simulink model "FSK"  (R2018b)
settings: Solver=VariableStepAuto  StartTime=0.0  StopTime=20  FixedStep=1e-5  RelTol=1e-3
libraries: commdigbbndfm2 x2, commchan3 x1, commrandsrc3 x1, dspsrcs4 x1

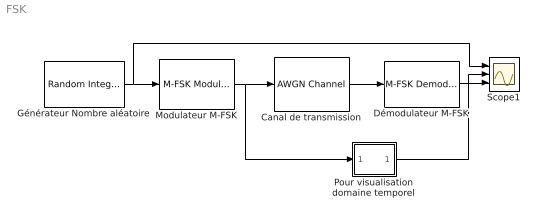
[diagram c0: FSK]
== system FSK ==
  Canal de transmission : commchan3/AWGN Channel  InputProcessing=Columns as channels (frame based)  seed=67  noiseMode="Signal to noise ratio  (Eb/No)"  EbNodB=10  EsNodB=10  SNRdB=10  bitsPerSym=1  Ps=1  Tsym=1  variance=1
  Démodulateur M-FSK : commdigbbndfm2/M-FSK Demodulator Baseband  M=4  OutType=Integer  Dec=Binary  freqSep=10  numSamp=100000  RateOptions=Enforce single-rate processing  outDataType=double
  Générateur Nombre aléatoire : commrandsrc3/Random Integer Generator  SetSize=4  SeedSource=Auto  Seed=0  SampleTime=1  SamplesPerFrame=1  OutputDataType=double  SimulateUsing=Interpreted execution
  Modulateur M-FSK : commdigbbndfm2/M-FSK Modulator Baseband  M=4  InType=Integer  Enc=Binary  freqSep=10  phaseType=Continuous  numSamp=100000  RateOptions=Enforce single-rate processing  outDataType=double
  Pour visualisation domaine temporel : Subsystem
  Scope1 : Scope  NumInputPorts=3
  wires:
  Modulateur M-FSK/1 -> Canal de transmission/1, Pour visualisation domaine temporel/1(In1)
  Canal de transmission/1 -> Démodulateur M-FSK/1
  Générateur Nombre aléatoire/1 -> Scope1/1, Modulateur M-FSK/1
  Démodulateur M-FSK/1 -> Scope1/3
  Pour visualisation domaine temporel/1(Out1) -> Scope1/2

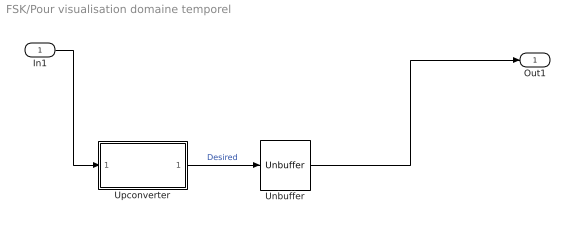
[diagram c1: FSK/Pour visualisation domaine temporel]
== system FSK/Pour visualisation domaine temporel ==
  In1 : Inport
  Unbuffer : Unbuffer
  Upconverter : Subsystem
  Out1 : Outport
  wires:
  Upconverter/1(Out) -> Unbuffer/1  "Desired"
  In1/1 -> Upconverter/1(In)
  Unbuffer/1 -> Out1/1

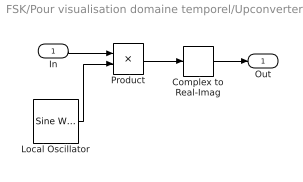
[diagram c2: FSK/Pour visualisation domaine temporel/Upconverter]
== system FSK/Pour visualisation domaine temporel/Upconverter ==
  In : Inport
  Complex to Real-Imag : ComplexToRealImag  Output=Real
  Local Oscillator : dspsrcs4/Sine Wave  Amplitude=1  Frequency=20  Phase=0  SampleMode=Discrete  OutComplex=Complex  CompMethod=Trigonometric fcn  TableSize=Speed  SampleTime=1/100000  SamplesPerFrame=100000  ResetState=Restart at time zero  OutputFrames=off  dataType=double  wordLen=16  udDataType=sfix(16)  fracBitsMode=Best precision  numFracBits=15  OutDataTypeStr=double  LastOutDataTypeStr=double
  Product : Product
  Out : Outport
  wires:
  Complex to Real-Imag/1 -> Out/1
  Product/1 -> Complex to Real-Imag/1
  Local Oscillator/1 -> Product/2
  In/1 -> Product/1
